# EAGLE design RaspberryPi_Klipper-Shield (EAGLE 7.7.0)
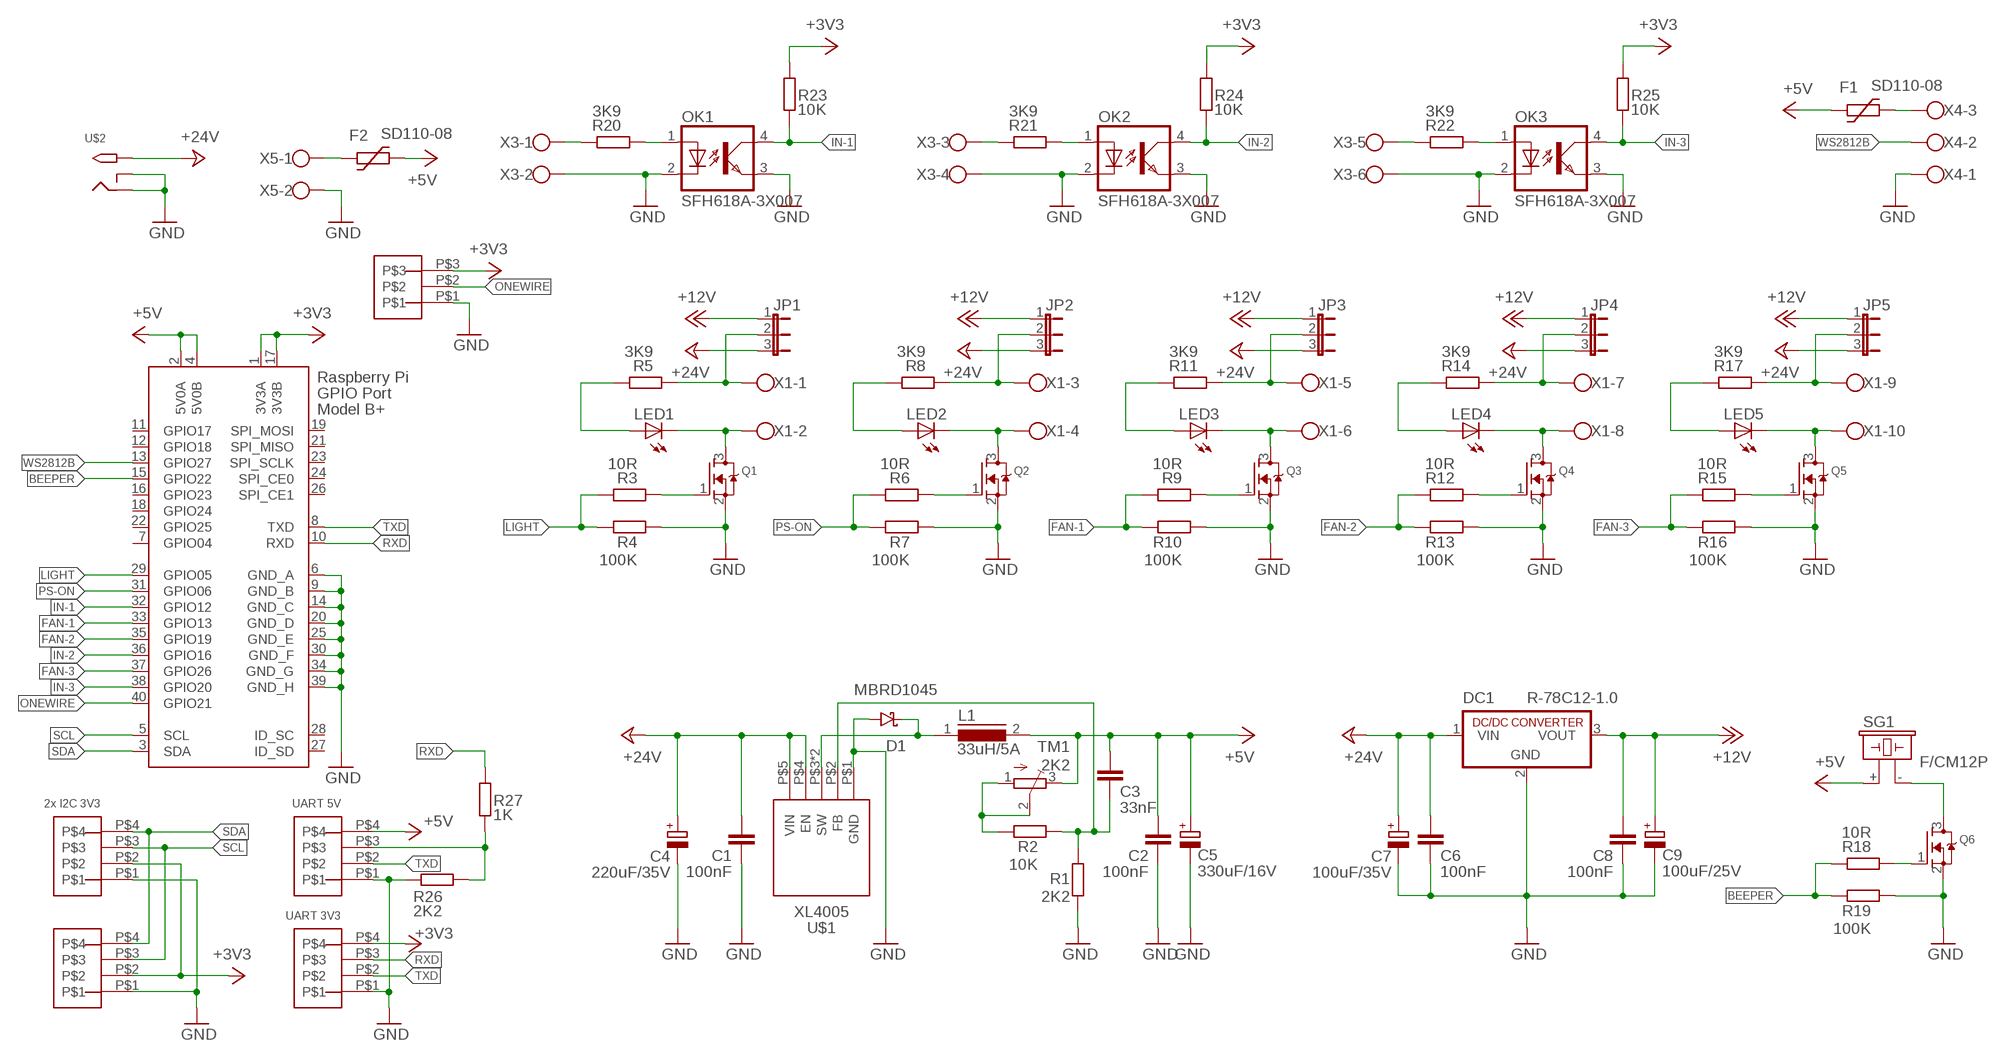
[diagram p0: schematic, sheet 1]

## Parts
C1  100nF  C-EUC1206  [C1206]
C2  100nF  C-EUC1206  [C1206]
C3  33nF  C-EUC1206  [C1206]
C4  220uF/35V  CPOL-EU153CLV-0605  [153CLV-0605]
C5  330uF/16V  CPOL-EU153CLV-0605  [153CLV-0605]
C6  100nF  C-EUC1206  [C1206]
C7  100uF/35V  CPOL-EU153CLV-0605  [153CLV-0605]
C8  100nF  C-EUC1206  [C1206]
C9  100uF/25V  CPOL-EU153CLV-0605  [153CLV-0605]
D1  MBRD1045  50WQ10FN  [TO-252-COMMON-PINS]
DC1  R-78C12-1.0  [SIP3]
F1  SD110-08  1812L  [1812L]
F2  SD110-08  1812L  [1812L]
JP1  JP2E  [JP2]
JP2  JP2E  [JP2]
JP3  JP2E  [JP2]
JP4  JP2E  [JP2]
JP5  JP2E  [JP2]
L1  33uH/5A  DR127  [DR127]
LED1  LEDCHIPLED_1206  [CHIPLED_1206]
LED2  LEDCHIPLED_1206  [CHIPLED_1206]
LED3  LEDCHIPLED_1206  [CHIPLED_1206]
LED4  LEDCHIPLED_1206  [CHIPLED_1206]
LED5  LEDCHIPLED_1206  [CHIPLED_1206]
OK1  SFH618A-3X007  [SMD4-7]
OK2  SFH618A-3X007  [SMD4-7]
OK3  SFH618A-3X007  [SMD4-7]
Q1  MOSFET-NREFLOW  [SOT23]
Q2  MOSFET-NREFLOW  [SOT23]
Q3  MOSFET-NREFLOW  [SOT23]
Q4  MOSFET-NREFLOW  [SOT23]
Q5  MOSFET-NREFLOW  [SOT23]
Q6  MOSFET-NREFLOW  [SOT23]
R1  2K2  R-EU_R1206  [R1206]
R2  10K  R-EU_R1206  [R1206]
R3  10R  R-EU_R1206  [R1206]
R4  100K  R-EU_R1206  [R1206]
R5  3K9  R-EU_R1206  [R1206]
R6  10R  R-EU_R1206  [R1206]
R7  100K  R-EU_R1206  [R1206]
R8  3K9  R-EU_R1206  [R1206]
R9  10R  R-EU_R1206  [R1206]
R10  100K  R-EU_R1206  [R1206]
R11  3K9  R-EU_R1206  [R1206]
R12  10R  R-EU_R1206  [R1206]
R13  100K  R-EU_R1206  [R1206]
R14  3K9  R-EU_R1206  [R1206]
R15  10R  R-EU_R1206  [R1206]
R16  100K  R-EU_R1206  [R1206]
R17  3K9  R-EU_R1206  [R1206]
R18  10R  R-EU_R1206  [R1206]
R19  100K  R-EU_R1206  [R1206]
R20  3K9  R-EU_R1206  [R1206]
R21  3K9  R-EU_R1206  [R1206]
R22  3K9  R-EU_R1206  [R1206]
R23  10K  R-EU_R1206  [R1206]
R24  10K  R-EU_R1206  [R1206]
R25  10K  R-EU_R1206  [R1206]
R26  2K2  R-EU_R1206  [R1206]
R27  1K  R-EU_R1206  [R1206]
SG1  F/CM12P  [F/CM12P]
TM1  2K2  TRIMPOTTC33X  [TC33X]
U$1  XL4005  [TO263-5L]
U$2  2.1MMJACKTHM  [PJ-102A]
U$3  4_PIN_JST-XH  [4_PIN_JST-XH]
U$4  4_PIN_JST-XH  [4_PIN_JST-XH]
U$5  4_PIN_JST-XH  [4_PIN_JST-XH]
U$6  4_PIN_JST-XH  [4_PIN_JST-XH]
U$7  3_PIN_JST-XH  [3_PIN_JST-XH]
X1  AK550/10  [AK550/10]
X2  RASPI_BOARD_B+#_E4  [RASPI_BOARD_B+_EDGES_4DRILL]
X3  AK550/6  [AK550/6]
X4  AK550/3  [AK550/3]
X5  AK550/2  [AK550/2]

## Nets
+3V3: R23.1 R24.1 R25.1 U$3.P$2 U$4.P$2 U$6.P$4 U$7.P$3 X2.1(3V3A) X2.17(3V3B)
+5V: C2.1 C3.1 C5.+ F1.P$1 F2.P$2 L1.2 SG1.+ TM1.3(E) U$5.P$4 X2.2(5V0A) X2.4(5V0B)
+12V: C8.1 C9.+ DC1.3(VOUT) JP1.1 JP2.1 JP3.1 JP4.1 JP5.1
+24V: C1.1 C4.+ C6.1 C7.+ DC1.1(VIN) JP1.3 JP2.3 JP3.3 JP4.3 JP5.3 U$1.P$4(EN) U$1.P$5(VIN) U$2.TIP
BEEPER: R18.2 R19.2 X2.15(GPIO22)
FAN-1: R9.2 R10.2 X2.33(GPIO13)
FAN-2: R12.2 R13.2 X2.35(GPIO19)
FAN-3: R15.2 R16.2 X2.37(GPIO26)
GND: C1.2 C2.2 C4.- C5.- C6.2 C7.- C8.2 C9.- D1.PINS(ANODE) DC1.2(GND) OK1.2(C) OK1.3(EMIT) OK2.2(C) OK2.3(EMIT) OK3.2(C) OK3.3(EMIT) Q1.2(S) Q2.2(S) Q3.2(S) Q4.2(S) Q5.2(S) Q6.2(S) R1.1 R4.1 R7.1 R10.1 R13.1 R16.1 R19.1 R26.2 U$1.P$1(GND) U$2.RING U$2.RING_SW U$3.P$1 U$4.P$1 U$5.P$1 U$6.P$1 U$7.P$1 X2.6(GND_A) X2.9(GND_B) X2.14(GND_C) X2.20(GND_D) X2.25(GND_E) X2.30(GND_F) X2.34(GND_G) X2.39(GND_H) X3.2 X3.4 X3.6 X4.1 X5.2
IN-1: OK1.4(COL) R23.2 X2.32(GPIO12)
IN-2: OK2.4(COL) R24.2 X2.36(GPIO16)
IN-3: OK3.4(COL) R25.2 X2.38(GPIO20)
LIGHT: R3.2 R4.2 X2.29(GPIO05)
N$1: R2.2 TM1.1(A) TM1.2(S)
N$2: Q1.1(G) R3.1
N$3: D1.PAD(CATHODE) L1.1 U$1.P$3(SW) U$1.P$6(SW)
N$4: LED1.C Q1.3(D) X1.2
N$5: C3.2 R1.2 R2.1 U$1.P$2(FB)
N$6: F1.P$2 X4.3
N$7: LED1.A R5.2
N$8: JP1.2 R5.1 X1.1
N$9: Q2.1(G) R6.1
N$10: OK1.1(A) R20.1
N$11: LED2.C Q2.3(D) X1.4
N$12: LED2.A R8.2
N$13: JP2.2 R8.1 X1.3
N$14: Q3.1(G) R9.1
N$15: R26.1 R27.2 U$5.P$3
N$16: LED3.C Q3.3(D) X1.6
N$17: LED3.A R11.2
N$18: JP3.2 R11.1 X1.5
N$19: Q4.1(G) R12.1
N$20: F2.P$1 X5.1
N$21: LED4.C Q4.3(D) X1.8
N$22: LED4.A R14.2
N$23: JP4.2 R14.1 X1.7
N$24: Q5.1(G) R15.1
N$25: Q6.1(G) R18.1
N$26: LED5.C Q5.3(D) X1.10
N$27: LED5.A R17.2
N$28: JP5.2 R17.1 X1.9
N$29: OK2.1(A) R21.1
N$30: OK3.1(A) R22.1
N$31: Q6.3(D) SG1.-
N$33: R20.2 X3.1
N$34: R21.2 X3.3
N$35: R22.2 X3.5
ONEWIRE: U$7.P$2 X2.40(GPIO21)
PS-ON: R6.2 R7.2 X2.31(GPIO06)
RXD: R27.1 U$6.P$3 X2.10(RXD)
SCL: U$3.P$3 U$4.P$3 X2.5(SCL)
SDA: U$3.P$4 U$4.P$4 X2.3(SDA)
TXD: U$5.P$2 U$6.P$2 X2.8(TXD)
WS2812B: X2.13(GPIO27) X4.2
Unconnected: X2.7(GPIO04) X2.11(GPIO17) X2.12(GPIO18) X2.16(GPIO23) X2.18(GPIO24) X2.19(SPI_MOSI) X2.21(SPI_MISO) X2.22(GPIO25) X2.23(SPI_SCLK) X2.24(SPI_CE0) X2.26(SPI_CE1) X2.27(ID_SD) X2.28(ID_SC)

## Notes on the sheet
- 2x I2C 3V3 | UART 5V
- UART 3V3

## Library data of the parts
C1-C3 C6 C8 = rcl:C-EU: CAPACITOR, European symbol
C4 C5 C7 C9 = rcl:CPOL-EU: POLARIZED CAPACITOR, European symbol
D1 = m_diode:50WQ10FN: 5 Amp Schottky Rectifier
DC1 = dc-dc-converter:R-78C*-1.0: INNOLINE DC/DC-Converter 1.0 AMP SIP3 Single Output Source: Data sheet
F1 F2 = ptc-littlefuse:1812L
JP1-JP5 = jumper:JP2E: JUMPER
L1 = inductors:DR127: High Power Density, High Efficiency, Shielded Inductors
LED1-LED5 = adafruit:LED: LED
OK1-OK3 = optocoupler:SFH618?*: Optocoupler, Phototransistor Output, Low Input Current Source: Data sheet; OC_FARNELL: unknown; OC_NEWARK: unknown
Q1-Q6 = adafruit:MOSFET-N: N-Channel Mosfet 2N7002E - 60V 260mA SOT23 [Digikey: 2N7002ET1GOSTR-ND] - REEL BSH103 - 30V 850mA SOT23 [Digikey: 568-5013-1-ND]
R1-R27 = rcl:R-EU_: RESISTOR, European symbol
SG1 = buzzer:F/CM12P: BUZZER; OC_FARNELL: unknown; OC_NEWARK: unknown
TM1 = adafruit:TRIMPOT: SMT trimmer potentiometer part number TC33X http://www.ladyada.net/library/eagle
U$1 = XL4005:XL4005
U$2 = adafruit:2.1MMJACK: 2.1mm x 5.5mm THM DC jack with internal switch. Digikey part #PJ-102A, 4UCON part #05537 2.1mm x 5.5mm SMT DC jack with internal switch. Digikey part #PJ-002A-SMT, 4UCON part #03267 By microbuilder.eu & adafruit.com
U$3-U$6 = JST-XH_HEADERS:4_PIN_JST-XH
U$7 = JST-XH_HEADERS:3_PIN_JST-XH
X1 = con-ptr500+:AK550/10: CONNECTOR
X2 = raspberrypi_bastelstube_v13:RASPI_BOARD_B+#: Raspberry Pi GPIO connector with markings for the outer dimensions of the Raspberry Pi board model B+ with different sets of drill holes or mounting pads All pins connected
X3 = con-ptr500+:AK550/6: CONNECTOR
X4 = con-ptr500+:AK550/3: CONNECTOR
X5 = con-ptr500+:AK550/2: CONNECTOR

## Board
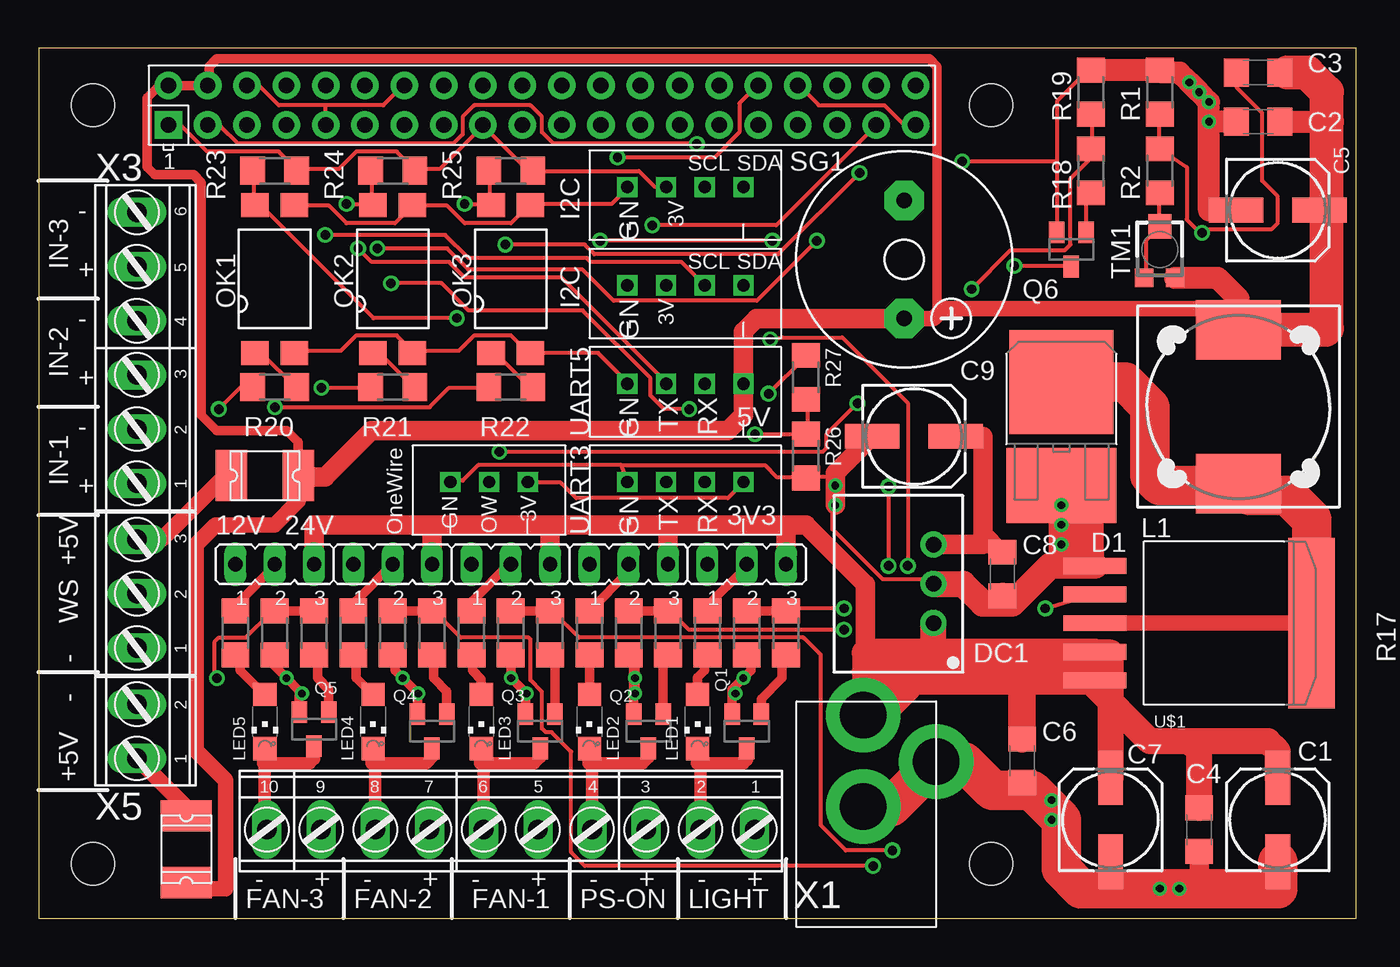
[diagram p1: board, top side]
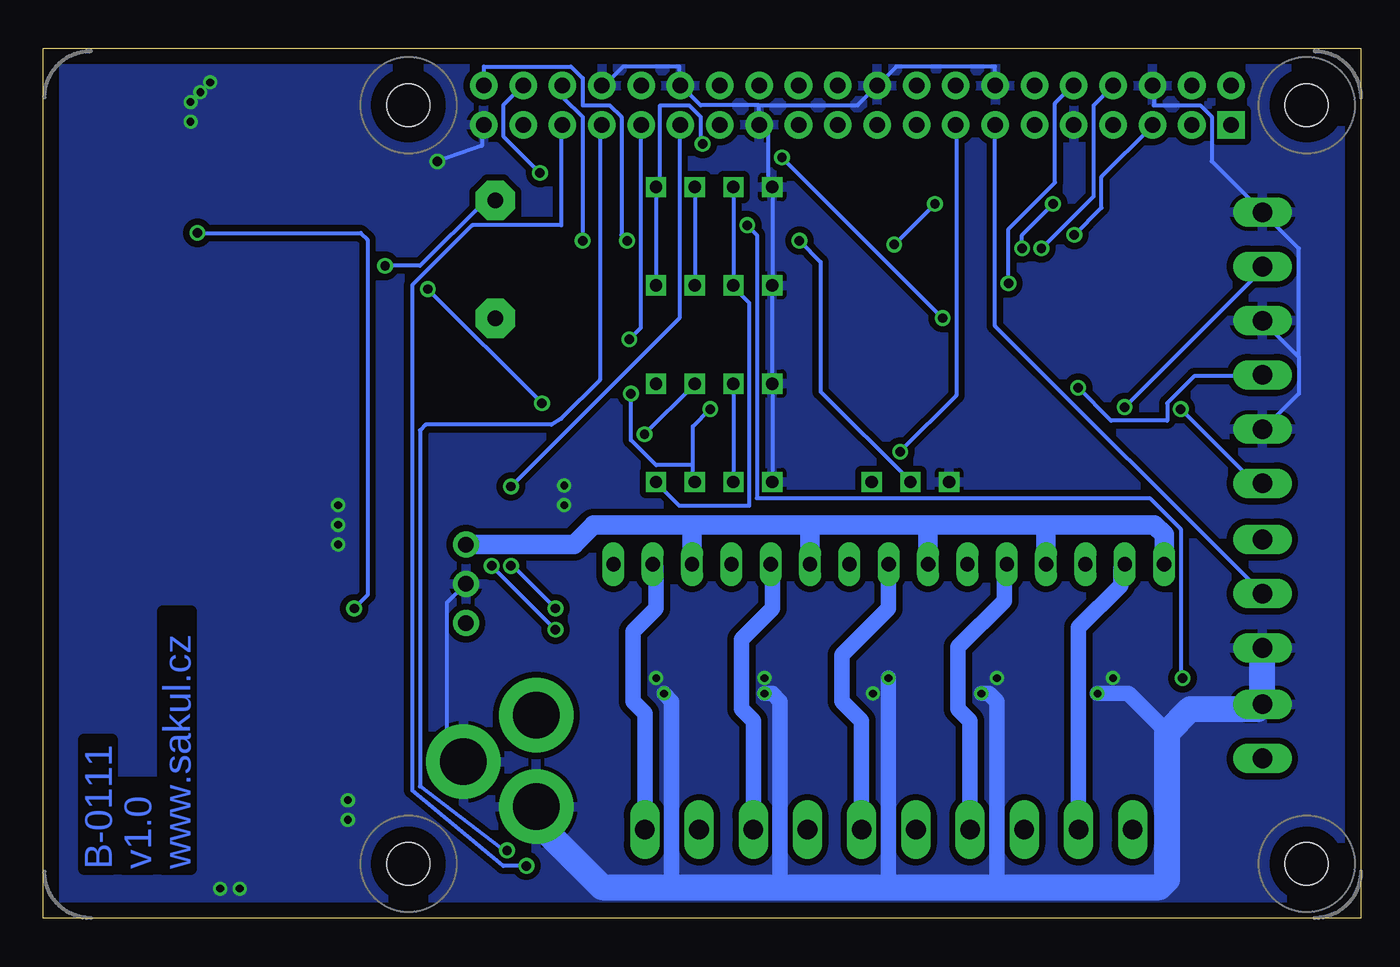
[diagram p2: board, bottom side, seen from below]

Size 85.07 x 56.19 mm. Coordinates in mm from the lower left corner, seen from the top.
Outline: 0,0 85.07,0 85.07,56.19 0,56.19 0,0
Copper layers (1*16): Top 0.035mm / dielectric 1.5mm / Bottom 0.035mm
Design rules "default": minimum track width 10mil, minimum drill 24mil, track to track 8mil, track to pad 8mil, pad to pad 8mil, via to via 8mil, smd to smd 8mil, copper to edge 40mil, drill to drill 8mil, minimum pad ring 10mil, minimum via ring 8mil, stop-mask expansion 4mil, vias tented up to drill 0mil, thermal gap 10mil

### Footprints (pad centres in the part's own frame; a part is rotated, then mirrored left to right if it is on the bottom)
C1206 = smd 1.6 x 1.8: 1 -1.4,0; 2 1.4,0
153CLV-0605 = smd 3.5 x 1.6: + 2.7,0; - -2.7,0
TO-252-COMMON-PINS = smd 6.7 x 6.7: PAD -0.96,0 | smd 4.826 x 7.112: PINS 5.715,0
SIP3 = drill 1 pad 1.676: 1 -2.54,0; 2 0,0; 3 2.54,0
1812L = smd 2.03 x 3.3: P$1 -2.16,0; P$2 2.16,0
JP2 = drill 0.914 long: 1 -2.54,0; 2 0,0; 3 2.54,0
DR127 = smd 3.85 x 5.5: 1 -4.975,0; 2 4.975,0
CHIPLED_1206 = smd 1.5 x 1.5: A 0,-1.75; C 0,1.75
SMD4-7 = smd 1.78 x 1.55: 1 -1.27,-4.77; 2 1.27,-4.77; 3 1.27,4.77; 4 -1.27,4.77
SOT23 = smd 1 x 1.4: 1 -0.95,-1.1; 2 0.95,-1.1; 3 0,1.1
R1206 = smd 1.6 x 1.803: 1 -1.422,0; 2 1.422,0
F/CM12P = drill 1.016 pad 2.54 octagon: + 3.81,0; - -3.81,0
TC33X = smd 1.2 x 1.2: 1 -1,-1.825; 3 1,-1.825 | smd 1.5 x 1.6: 2 0,1.5
TO263-5L = smd 1.02 x 4.06: P$1 -3.7,-8; P$2 -1.85,-8; P$3 0,-8; P$4 1.85,-8; P$5 3.7,-8 | smd 11 x 3: P$6 0,6
PJ-102A = drill 3 pad 4.8: RING 0.1,-3.39; RING_SW -4.6,-6.29; TIP 0.1,-9.29
4_PIN_JST-XH = drill 0.8 square: P$1 2.45,3.4; P$2 4.95,3.4; P$3 7.45,3.4; P$4 9.95,3.4
3_PIN_JST-XH = drill 0.8 square: P$1 2.45,3.4; P$2 4.95,3.4; P$3 7.45,3.4
AK550/10 = drill 1.27 long: 1 -15.75,0; 2 -12.25,0; 3 -8.75,0; 4 -5.25,0; 5 -1.75,0; 6 1.75,0; 7 5.25,0; 8 8.75,0; 9 12.25,0; 10 15.75,0
RASPI_BOARD_B+_EDGES_4DRILL = drill 1 pad 1.778 square: 1 8.37,51.23 | drill 1 pad 1.778: 2 8.37,53.77; 3 10.91,51.23; 4 10.91,53.77; 5 13.45,51.23; 6 13.45,53.77; 7 15.99,51.23; 8 15.99,53.77; 9 18.53,51.23; 10 18.53,53.77; 11 21.07,51.23; 12 21.07,53.77; 13 23.61,51.23; 14 23.61,53.77; 15 26.15,51.23; 16 26.15,53.77; 17 28.69,51.23; 18 28.69,53.77; 19 31.23,51.23; 20 31.23,53.77; 21 33.77,51.23; 22 33.77,53.77; 23 36.31,51.23; 24 36.31,53.77; 25 38.85,51.23; 26 38.85,53.77; 27 41.39,51.23; 28 41.39,53.77; 29 43.93,51.23; 30 43.93,53.77; 31 46.47,51.23; 32 46.47,53.77; 33 49.01,51.23; 34 49.01,53.77; 35 51.55,51.23; 36 51.55,53.77; 37 54.09,51.23; 38 54.09,53.77; 39 56.63,51.23; 40 56.63,53.77 | hole 2.75: 3.5,3.5; 3.5,52.5; 61.5,3.5; 61.5,52.5
AK550/6 = drill 1.27 long: 1 -8.75,0; 2 -5.25,0; 3 -1.75,0; 4 1.75,0; 5 5.25,0; 6 8.75,0
AK550/3 = drill 1.27 long: 1 -3.5,0; 2 0,0; 3 3.5,0
AK550/2 = drill 1.27 long: 1 -1.75,0; 2 1.75,0

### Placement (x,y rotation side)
C1  74.93,5.71 270 top
C2  78.74,51.44 180 top
C3  78.74,54.61 180 top
C4  80.01,6.35 90 top
C5  80.01,45.72 0 top
C6  63.5,10.16 270 top
C7  69.22,6.35 90 top
C8  62.23,22.23 270 top
C9  56.52,31.11 0 top
D1  66.04,33.66 270 top
DC1  57.78,21.59 90 top
F1  14.61,28.57 180 top
F2  9.53,4.45 270 top
JP1  45.72,22.86 0 top
JP2  38.1,22.86 0 top
JP3  30.48,22.86 0 top
JP4  22.86,22.86 0 top
JP5  15.24,22.86 0 top
L1  77.47,33.02 90 top
LED1  42.55,12.7 180 top
LED2  35.56,12.7 180 top
LED3  28.57,12.7 180 top
LED4  21.59,12.7 180 top
LED5  14.61,12.7 180 top
OK1  15.24,41.27 0 top
OK2  22.86,41.27 0 top
OK3  30.48,41.27 0 top
Q1  45.72,12.06 180 top
Q2  39.37,12.06 180 top
Q3  32.38,12.06 180 top
Q4  25.4,12.06 180 top
Q5  17.78,12.2 180 top
Q6  66.67,43.18 180 top
R1  72.39,53.34 270 top
R2  72.39,48.26 270 top
R3  48.26,18.41 90 top
R4  45.72,18.41 90 top
R5  43.18,18.41 270 top
R6  40.64,18.41 90 top
R7  38.1,18.41 90 top
R8  35.56,18.41 270 top
R9  33.02,18.41 90 top
R10  30.48,18.41 90 top
R11  27.94,18.41 270 top
R12  25.4,18.41 90 top
R13  22.86,18.41 90 top
R14  20.32,18.41 270 top
R15  17.78,18.41 90 top
R16  15.24,18.41 90 top
R17  12.7,18.41 270 top
R18  67.94,48.26 90 top
R19  67.94,53.34 270 top
R20  15.24,34.29 180 top
R21  22.86,34.29 180 top
R22  30.48,34.29 180 top
R23  15.24,48.26 180 top
R24  22.86,48.26 180 top
R25  30.48,48.26 180 top
R26  49.53,29.84 270 top
R27  49.53,34.92 270 top
SG1  55.88,42.55 270 top
TM1  72.39,43.18 0 top
U$1  76.2,19.05 270 top
U$2  53.34,3.81 180 top
U$3  35.56,37.47 0 top
U$4  35.56,43.81 0 top
U$5  35.56,31.11 0 top
U$6  35.56,24.77 0 top
U$7  24.13,24.77 0 top
X1  30.48,5.71 180 top
X2  0,0 0 top
X3  6.35,36.83 90 top
X4  6.35,20.95 90 top
X5  6.35,12.06 90 top

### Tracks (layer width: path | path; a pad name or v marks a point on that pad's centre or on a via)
+3V3
  Top 0.254: X2.1 8.38,51.12 9.25,51.12 10.88,49.5 15.5,49.5 16.62,48.38 R23.1 16.75,48.38 19.38,48.38 20.5,49.5 23.12,49.5 24.25,48.38 R24.1 24.38,48.38 25.88,48.38 28.62,51.12 X2.17 28.75,51.12 31.5,48.38 31.88,48.38 R25.1 32,48.25 38.75,48.25 39.75,47.25 40.5,47.25 U$4.P$2 | U$7.P$3 31.62,28.12 33.71,28.12 34.71,27.12 44.5,27.12 45.5,28.12 U$6.P$4
  Bottom 0.254: U$4.P$2 40.5,47.12 U$3.P$2 40.5,40.75 39.5,39.75 39.5,26.62 44,26.62 45.5,28.12 U$6.P$4
+5V
  Top 0.254: 45.5,34.62 U$5.P$4 | 45.5,36.62 45.51,37.89
  Top 0.406: 58.42,39.37 58.42,39.58 58,39
  Top 0.61: 58,39 58,55 57.5,55.5 11.5,55.5 11,55 11,53.86 X2.4 X2.2 | F1.P$1 16.77,30.73 16,31.5 11.5,31.5 10.5,32.5 10.5,47.5 10,48 7.5,48 7,48.5 7,53 8,54 8.5,53.5
  Top 1.016: F1.P$1 16.77,26.93 15.24,25.4 11.43,25.4 10.16,24.13 10.16,10.79 12.06,8.89 12.06,1.91 9.9,1.91 F2.P$2 | SG1.+ 57.78,38.73 58.42,39.37 77.47,39.37
  Top 1.27: 45.51,37.89 46.35,38.73 SG1.+ | 45.5,37.63 45.5,36.62 45.5,34.62 45.5,32.5 44.5,31.5 21.5,31.5 18.5,28.5 16.84,28.5 F1.P$1
  Top 1.422: C2.1 83.19,51.44 | C3.1 81.28,54.61 | C5.+ 83.19,45.72 | TM1.3 76.12,41.35 77.47,40.01 77.47,39.37 L1.2
  Top 2.184: L1.2 83.08,37.99 83.19,38.1 83.19,45.72 83.19,51.44 83.19,53.34 81.92,54.61 81.28,54.61 80.64,54.61
+12V
  Top 1.27: C9.+ 60.96,31.11 60.96,24.77 | 60.96,24.77 60.96,24.13 DC1.3 | C8.1 62.1,23.62 60.96,24.77
  Bottom 1.27: DC1.3 50.8,24.13 49.53,25.4 43.18,25.4 | 43.18,25.4 35.56,25.4 | 35.56,25.4 27.94,25.4 | 27.94,25.4 20.32,25.4 | 20.32,25.4 13.34,25.4 12.7,24.77 JP5.1 | JP4.1 20.32,25.4 | JP3.1 27.94,25.4 | JP2.1 35.56,25.4 | JP1.1 43.18,25.4
+24V
  Top 1.27: 53.4,17.2 53.4,21.54 49.53,25.4 48.26,25.4 | 48.26,25.4 40.64,25.4 | 40.64,25.4 33.02,25.4 | 33.02,25.4 25.4,25.4 | 25.4,25.4 17.78,25.4 JP5.3 | JP4.3 25.4,25.4 | JP3.3 33.02,25.4 | JP2.3 40.64,25.4 | JP1.3 48.26,25.4
  Top 1.676: 53.4,17.2 U$1.P$4 68.25,17.14 69.22,17.14 C7.+ | 53.4,17.2 53.34,17.14 53.34,15.88 | 53.34,15.88 53.34,13.34 | 53.34,13.34 53.34,13.2 U$2.TIP | 53.4,17.2 53.4,15.93 53.34,15.88 | 53.34,15.88 63.5,15.88 67.94,15.88 | 67.94,15.88 67.94,17.14 | 67.94,15.88 67.94,15.61 | 67.94,15.61 U$1.P$5 68.09,15.24 67.94,15.24 | 67.94,15.61 67.94,15.24 | 67.94,15.24 55.24,15.24 53.34,13.34 | 53.34,13.34 54.61,13.34 57.78,16.51 DC1.1 | C4.+ 80.01,10.79 79.38,11.43 74.3,11.43 | 74.3,11.43 71.75,11.43 67.94,15.24 | C1.1 74.93,10.79 74.3,11.43
  Top 1.778: C6.1 63.5,15.88
BEEPER  (via drill 0.61)
  Top 0.254: R19.2 68,51.88 68,49.75 R18.2 67.88,49.62 67.88,49 66.62,47.75 66.62,43.5 66.25,43.12 62.75,43.12 v60.25,40.62 | v52.88,33.25 50.88,31.25 50.88,30.38 50.62,30.12 v29.75,30.12
  Bottom 0.254: v52.88,33.25 v60.25,40.62 | v29.75,30.12 26.12,33.75 26.12,51.12 X2.15
FAN-1  (via drill 0.61)
  Top 0.254: v55.12,4.38 52.12,4.38 50.5,6 50.5,17 49.38,18.12 34.88,18.12 33.25,19.75 R9.2
  Top 0.61: R10.2 R9.2
  Bottom 0.254: X2.33 49.12,51.12 49.12,34.75 51.62,32.25 52.26,31.88 60.38,31.88 60.75,31.5 60.75,8.5 55.5,4.5 55.38,4.38 v55.12,4.38
FAN-2  (via drill 0.61)
  Top 0.254: v53.88,3.38 35.25,3.38 34.38,4.25 34.38,10.75 33.12,12 32.75,12 32.5,12.25 32.5,14.62 31.75,15.38 31.75,18 31.62,18.12 27.25,18.12 25.62,19.75 R12.2
  Top 0.61: R13.2 R12.2
  Bottom 0.254: X2.35 51.62,51.12 51.62,44.75 57.38,44.75 61.25,40.88 61.25,8.25 55.38,3.38 v53.88,3.38
FAN-3  (via drill 0.61)
  Top 0.254: v11.5,15.5 11.38,15.62 11.38,17.88 11.62,18.12 13.38,18.12 15,19.75 R16.2 | v39.62,44.75 47.62,44.75 54,51.12 X2.37
  Top 0.61: R16.2 R15.2
  Bottom 0.254: v11.5,15.5 11.62,15.62 11.62,25.12 13.62,27.12 39,27.12 39,44.12 v39.62,44.75
GND  (via drill 0.5, 0.61)
  Top 0.254: 53.75,31 C9.- | DC1.2 57,21.88 54.5,21.88 51.25,25.12 51.25,28.5 49.62,28.5 R26.2 49.5,28.5 47.63,28.5 46.88,29.25 37.63,29.25 | 37.63,29.25 28.38,29.25 27.38,28.25 26.62,28.25 U$7.P$1 | 37.63,29.25 38,28.25 U$6.P$1 | OK1.2 16.62,36.62 19.5,36.62 20.5,37.62 23.12,37.62 24.12,36.62 OK2.2 24.25,36.62 27.12,36.62 28.12,37.62 30.5,37.62 31.62,36.5 OK3.2 36.12,36.5 38,34.62 U$5.P$1 | 18.5,52.5 22.25,52.5 23.5,53.75 X2.14 | 18.62,51.25 X2.9 18.5,51.26 18.5,52.5 | 18.5,52.5 15.5,52.5 14.25,53.75 13.5,53.75 X2.6 | 65.75,48.88 65.75,52.75 67.62,54.62 R19.1 | 65.75,48.88 65.75,44.38 Q6.2 | OK1.3 16.62,46 18.75,46 19.88,44.88 23,44.88 24.12,46 OK2.3 24.25,46 26.38,46 27.5,44.88 30.5,44.88 31.62,46 OK3.3 31.75,46.12 37,46.12 38,47.12 U$4.P$1 | X2.39 56.62,51.25 55.88,51.25 54.62,52.5 50.38,52.5 49.12,53.75 X2.34 | v59.62,48.88 65.75,48.88
  Top 0.61: Q5.2 16.83,14.5 | 16.83,14.5 16.83,14.67 v16,15.5 15,16.5 15,16.75 R16.1 | Q4.2 24.45,14.5 | 24.45,14.5 24.45,14.55 v23.5,15.5 23,16 23,16.85 R13.1 | Q3.2 31.43,14.56 | 31.43,14.56 v30.5,15.5 30.5,16.97 R10.1 | Q2.2 38.42,16.5 | 38.42,16.5 38.42,16.67 R7.1 | Q1.2 44.77,14.5 | 44.77,14.5 44.77,14.77 v45.5,15.5 46,16 46,16.71 R4.1 | 31.43,14.56 v31.5,14.5 | v24.5,14.5 24.45,14.5 | v17,14.5 16.83,14.5 | v45,14.5 44.77,14.5 | v38.5,14.5 v38.5,15.5 38.5,16.42 38.42,16.5
  Top 1.27: C6.2 63.5,8.26 | C7.- 69.22,1.91 | C1.2 74.93,1.91 | v51.44,27.94 v51.44,26.67 51.44,28.73 C9.-
  Top 1.422: C5.- 75.56,45.72 v75.56,51.44 | v75.56,51.44 v75.56,52.7 v74.93,53.34 v74.3,53.98 73.66,54.61 72.54,54.61 R1.1 R19.1 | C2.2 v75.56,51.44
  Top 1.676: DC1.2 59.69,21.59 60.96,20.32 62.23,20.32 | 62.23,20.32 62.87,20.32 65.3,22.75 67.31,22.75 | C8.2 62.23,20.32 | U$1.P$1 67.31,22.75 | D1.PINS v66.04,26.67 v66.04,25.4 v66.04,24.13 66.04,23.5 67.94,23.5 67.94,26.67 67.31,26.67 66.67,26.04 66.67,23.39 67.31,22.75
  Top 2.54: U$2.RING 55.04,7.2 U$2.RING_SW 59.75,10.1 61.59,8.26 63.5,8.26 64.14,8.26 66.04,6.35 66.04,3.17 67.31,1.91 69.22,1.91 v72.39,1.91 v73.66,1.91 74.93,1.91 80.01,1.91 C4.-
  Bottom 0.254: DC1.2 59,20.38 59,11.12 58,10.12 U$2.RING_SW | U$6.P$1 38,28.25 38,34.5 U$5.P$1 38,34.62 38,40.75 U$3.P$1 38,47.12 U$4.P$1 38.12,47.25 38.25,47.38 38.25,50.62 38.75,51.12 X2.25 38.88,51.25 38.88,52.5 | 4,36.25 4,33.88 6.25,31.62 X3.2 | 4,36.25 6.25,38.5 X3.4 | 4,36.25 4,43.25 6.25,45.5 X3.6 6.38,45.62 9.62,48.88 9.62,51.75 10.38,52.5 13.38,52.5 13.38,53.75 X2.6 | X2.14 23.62,53.88 23.62,55 30,55 X2.20 32.5,52.5 38.88,52.5 | 38.88,52.5 42.62,52.5 43.88,53.75 X2.30 44,53.88 44,55 47.63,55 48.38,54.25 48.88,53.88 49,53.88 X2.34 | v59.62,48.88 56.75,49.88 56.75,51.12 X2.39
  Bottom 1.016: v17,14.5 15,14.5 12.5,12 | v24.5,14.5 24,14.5 23.5,14 23.5,2 | v30.5,15.5 30.5,2 | v38.5,14.5 38,14.5 37.5,14 37.5,2 | 44.5,2 44.5,14 v45,14.5
  Bottom 1.676: U$2.RING 53.24,6.24 49,2 44.5,2 37.5,2 30.5,2 23.5,2 13,2 12.5,2.5 12.5,12 11,13.5 6.67,13.5 X5.2 X4.1
  other vias: 65.41,7.62 65.41,6.35
  pour Bottom (isolate 0.406): 0,56 85,56 85,0 0,0
IN-1  (via drill 0.61)
  Top 0.254: R23.2 13.88,48.25 13.88,46.12 OK1.4 14,46 14.38,46 21.62,38.75 v27,38.75 | v37.38,49.12 43.62,49.12 45.25,50.75 45.25,52.62 46.38,53.75 X2.32
  Bottom 0.254: v37.38,49.12 v27,38.75
IN-2  (via drill 0.61)
  Top 0.254: R24.2 21.5,48.25 21.5,46.12 OK2.4 21.38,46.12 v19.88,46.12 | v21.88,43.25 26.38,43.25 27.75,41.88 35.12,41.88 37.12,39.88 46.38,39.88 v50.25,43.75
  Bottom 0.254: v19.88,46.12 21.88,44.12 v21.88,43.25 | v50.25,43.75 50.25,51.75 51.5,53 51.5,53.75 X2.36
IN-3  (via drill 0.61)
  Top 0.254: R25.2 29.12,48.25 29.12,46.12 OK3.4 29,46.12 v27.5,46.12 | v30.12,43.5 35.25,43.5 35.88,42.88 47.75,42.88 v53,48.12
  Bottom 0.254: v30.12,43.5 v27.5,46.12 | v53,48.12 55.38,50.5 55.38,52.5 54.12,53.75 X2.38
LIGHT  (via drill 0.61)
  Top 0.254: v52,20 48.5,20 R3.2 | v54.88,27.88 v54.88,22.75
  Top 0.61: R4.2 R3.2
  Bottom 0.254: v52,20 54.75,22.75 v54.88,22.75 | v54.88,27.88 44,38.75 44,51.12 X2.29
N$1
  Top 0.254: TM1.1 71.5,41.38 71.5,43.75 72.38,44.62 TM1.2 72.38,44.75 72.38,46.75 R2.2
N$2
  Top 0.61: Q1.1 46.67,14.17 48,15.5 48,16.73 R3.1
N$3
  Top 1.016: U$1.P$3 U$1.P$6
  Top 2.54: U$1.P$6 82.2,25.75 80.64,27.3 78.21,27.3 L1.1 77.36,27.94 72.39,27.94 71.75,28.57 71.75,33.02 70.16,34.62 D1.PAD
N$4
  Top 0.813: Q1.3 45.72,10.22 45.5,10 42.5,10 42.5,10.9 LED1.C 42.73,10.77 X1.2
N$5  (via drill 0.61)
  Top 0.254: 74.75,44.5 79.62,44.5 80,44.88 80,46.62 79,47.62 79,52 77.38,53.62 77.38,54.5 C3.2 | 74.75,44.5 74.12,45.12 74.12,48.5 72.5,49.62 R2.1 72.38,49.75 72.38,51.88 R1.2 | v65,20 68.25,21 U$1.P$2 | v75.12,44.25 75.25,44.38 74.75,44.5
  Bottom 0.254: v75.12,44.25 64.57,44.25 64.14,43.81 64.14,20.86 v65,20
N$6
  Top 1.016: F1.P$2 12.06,28.57 7.95,24.45 X4.3
N$7
  Top 0.61: LED1.A 42.55,15.54 43,16 43,16.81 R5.2
N$8
  Top 0.61: JP1.2 45.72,22.72 43,20 43.02,20 R5.1
  Bottom 1.016: X1.1 46.23,13.23 47,14 47,18.5 45.5,20 45.5,22.64 JP1.2
N$9
  Top 0.61: Q2.1 40.32,16.67 R6.1
N$10
  Top 0.254: OK1.1 14,36.5 14.38,36.5 16.62,34.25 R20.1
N$11
  Top 0.813: Q2.3 39.37,10.37 39,10 36,10 | 36,10 35.5,10 35.5,10.89 LED2.C | X1.4 35.73,9.73 36,10
N$12
  Top 0.61: LED2.A R8.2
N$13
  Top 0.61: JP2.2 38.1,22.38 R8.1
  Bottom 1.016: X1.3 39.23,12.73 40,13.5 40,18 38,20 38,22.76 JP2.2
N$14
  Top 0.61: Q3.1 33.34,16.68 R9.1
N$15  (via drill 0.61)
  Top 0.254: R27.2 49.62,33.5 49.62,31.38 R26.1 49.5,31.25 v46.25,31.25
  Bottom 0.254: v46.25,31.25 43.12,34.38 43.12,34.5 U$5.P$3
N$16
  Top 0.813: Q3.3 32.38,10.38 32,10 28.5,10 | 28.5,10 28.5,10.88 LED3.C | X1.6 28.73,9.77 28.5,10
N$17
  Top 0.61: LED3.A 28.57,15.43 28,16 28,16.93 R11.2
N$18
  Top 0.61: JP3.2 30.36,22.86 28,20.5 28,19.9 R11.1
  Bottom 1.016: X1.5 32.23,12.73 33.5,14 33.5,17 30.5,20 30.5,22.84 JP3.2
N$19
  Top 0.61: Q4.1 26.35,14.65 25.5,15.5 25.5,16.89 R12.1
N$20
  Top 1.016: F2.P$1 9.53,7.14 X5.1
N$21
  Top 0.813: Q4.3 25.4,10.4 25,10 22,10 | 22,10 21.5,10 21.5,10.86 LED4.C | X1.8 21.73,9.73 22,10
N$22
  Top 0.61: LED4.A 21.55,14.45 20.5,15.5 20.5,16.81 R14.2
N$23
  Top 0.61: JP4.2 20.5,20.5 20.5,20.02 R14.1
  Bottom 1.016: X1.7 25.23,12.73 26,13.5 26,17.5 23,20.5 23,22.72 JP4.2
N$24
  Top 0.61: Q5.1 18.73,14.77 18,15.5 18,16.77 R15.1
N$25
  Top 0.254: Q6.1 67.62,46.5 67.88,46.75 R18.1
N$26
  Top 0.813: Q5.3 17.78,10.28 17.5,10 14.5,10 14.5,10.85 LED5.C 14.61,5.84 X1.10
N$27
  Top 0.61: LED5.A 14.55,14.45 13,16 13,16.69 R17.2
N$28
  Top 0.61: JP5.2 15.24,22.74 13,20.5 13,20.14 R17.1
  Bottom 1.016: X1.9 18.23,18.77 15.5,21.5 15.5,22.6 JP5.2
N$29
  Top 0.254: OK2.1 21.62,36.5 22,36.5 24.25,34.25 R21.1
N$30
  Top 0.254: OK3.1 29.25,36.5 29.5,36.5 31.62,34.38 31.88,34.38 R22.1
N$31  (via drill 0.61)
  Top 0.254: v63,42.12 66.62,42.12 Q6.3
  Bottom 0.254: v63,42.12 60.75,42.12 56.62,46.25 56,46.25 SG1.-
N$33  (via drill 0.61)
  Top 0.254: v11.62,32.88 13,34.25 13.75,34.25 R20.2
  Bottom 0.254: v11.62,32.88 6.88,28.12 6.38,28.12 X3.1
N$34  (via drill 0.61)
  Top 0.254: v18.25,34.25 21.38,34.25 R21.2
  Bottom 0.254: v18.25,34.25 16.12,32.12 12.5,32.12 12.5,33.25 10.75,35 6.38,35 X3.3
N$35  (via drill 0.61)
  Top 0.254: v15.25,33 25.25,33 26.5,34.25 29,34.25 R22.2
  Bottom 0.254: v15.25,33 6.38,41.88 6.38,42 X3.5
ONEWIRE  (via drill 0.61)
  Top 0.254: v47.38,43.75 v36.25,43.75
  Bottom 0.254: v36.25,43.75 34.88,42.38 34.88,34 29.12,28.25 U$7.P$2 | v47.38,43.75 47.75,44.12 47.75,51.75 48.5,52.5 50.25,52.5 50.25,54.25 51,55 56.62,55 56.62,53.88 X2.40
PS-ON  (via drill 0.61)
  Top 0.254: v52,18.62 42,18.62 40.88,19.75 R6.2 | v56.12,22.75 56.12,33.27 51.9,37.5 48,37.5 v47.24,37.38
  Top 0.61: R7.2 R6.2
  Bottom 0.254: v56.12,22.75 v52,18.62 | v47.24,37.38 46.5,38.12 46.5,51.12 X2.31
RXD  (via drill 0.61)
  Top 0.254: v47.12,33.88 49.5,36.25 R27.1 | v22.75,41 26,41 27.75,39.25 35.12,39.25 39.5,34.88 39.5,33.75 40.38,32.88 v42.01,32.88
  Bottom 0.254: v47.12,33.88 47.12,30.88 45.5,29.25 43.12,29.25 | 43.12,29.25 43.12,28.25 U$6.P$3 | v22.75,41 22.75,44.5 19.75,47.5 19.75,52.62 18.62,53.75 X2.10 | v42.01,32.88 43.12,31.76 43.12,29.25
SCL  (via drill 0.61)
  Top 0.254: v18.5,44.12 26.25,44.12 27.75,42.62 35.38,42.62 35.62,42.38 41.5,42.38 U$3.P$3
  Bottom 0.254: U$3.P$3 43,47.12 U$4.P$3 | v18.5,44.12 16.75,45.88 16.75,47.88 13.5,51.12 X2.5
SDA  (via drill 0.61)
  Top 0.254: v42.5,50 33.25,50 32.5,50.75 32.5,51.75 31.75,52.5 28.12,52.5 27.38,51.75 27.38,50.62 26.75,50 12.88,50 11.75,51.12 11,51.12 X2.3
  Bottom 0.254: U$3.P$4 45.5,47.12 U$4.P$4 45.5,47.25 45.25,47.5 45.25,52.5 43.38,52.5 42.62,51.75 42.62,50.12 v42.5,50
TXD  (via drill 0.61)
  Top 0.254: v20.62,43.25 21.5,42.38 26.5,42.38 27.5,41.38 33.75,41.38 40.5,34.62 U$5.P$2
  Bottom 0.254: U$6.P$2 40.5,28.25 40.5,34.5 U$5.P$2 | v20.62,43.25 17.25,46.62 17.25,52.5 16,53.75 X2.8
WS2812B
  Bottom 0.254: X2.13 23.62,51.12 23.62,38.25 6.38,21 X4.2

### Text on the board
Bottom: www.sakul.cz | v1.0 | B-0111
tPlace: SCL | SDA | GN | 3V | - | I2C | IN-3 | SCL | SDA | + | GN | 3V | I2C | - | IN-2 | + | GN | TX | RX | 5V | - | UART5 | IN-1 | + | GN | OW | 3V | GN | TX | RX | +5V | 12V | 24V | OneWire | UART3 | 3V3 | WS | - | - | +5V | - | + | - | + | - | + | - | + | - | + | FAN-3 | FAN-2 | FAN-1 | PS-ON | LIGHT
